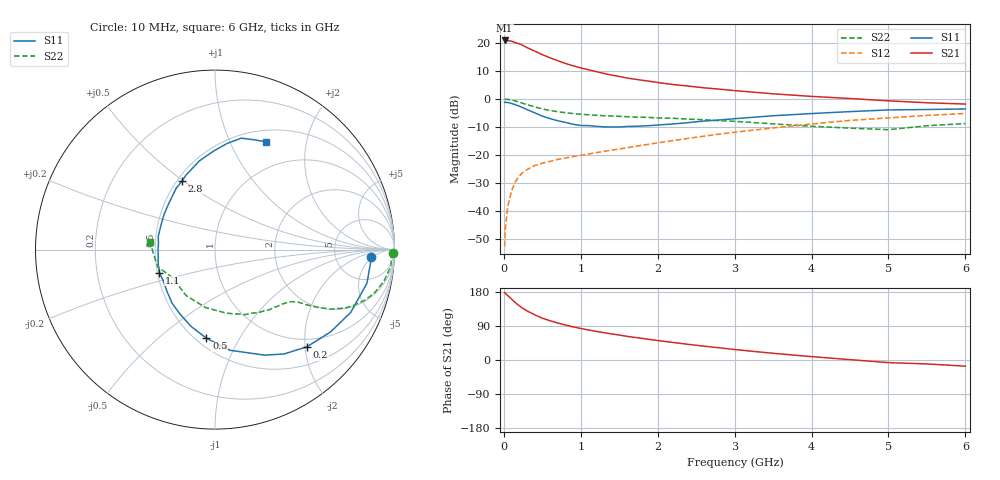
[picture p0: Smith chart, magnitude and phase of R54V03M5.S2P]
! SIEMENS Small Signal Semiconductors
! BFR183
! Si NPN RF Bipolar Junction Transistor in SOT23
! VCE = 4 V  IC = 3.5 mA
! Common Emitter S-Parameters:  May  1996
# GHz  S  MA  R  50
!  f  S11  S21  S12  S22
! GHz  MAG  ANG  MAG  ANG  MAG  ANG  MAG  ANG
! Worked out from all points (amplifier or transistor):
!   36 points, 10 MHz to 6 GHz, reference 50 ohm
!   highest |S21| = 20.8 dB at 10 MHz (marker M1)
!   |S21| within 3 dB of that: start of sweep to 337.5 MHz
!   unconditionally stable (mu >= 1): 1.211 GHz to 2.683 GHz
!   at 250 MHz: K = 0.33, MSG = 22.6 dB, |S12| = -26.1 dB
!   at 1.4 GHz: K = 1.05, MAG = 12.0 dB, |S12| = -18.2 dB
!   at 6 GHz: K = 0.88, MSG = 1.7 dB, |S12| = -5.2 dB
!   S11 on the Smith chart (normalised r, x): 10 MHz: 13, -4; 200 MHz: 0.84, -2.04; 500 MHz: 0.56, -0.74; 1.1 GHz: 0.51, -0.15; 2.8 GHz: 0.53, +0.49; 6 GHz: 0.64, +1.38
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0.01  0.8713 -2.6  11 178.2  0.0024 87.6  0.9932 -1.1
0.02  0.8698 -4.9  10.8 175.9  0.005 87.3  0.9833 -2.1
0.05  0.867 -12.5  10.9 170.2  0.0118 82.9  0.9842 -5.4
0.1  0.8333 -24.8  10.69 160.8  0.0233 77.3  0.9582 -10.5
0.15  0.7905 -35.5  10.04 151.3  0.0336 71.2  0.9224 -15.0
0.2  0.7453 -46.6  9.587 143.3  0.0422 66.9  0.8824 -18.6
0.25  0.6974 -56.5  8.943 135.9  0.0495 62.1  0.8341 -21.8
0.3  0.6494 -64.9  8.214 129.7  0.0553 59.7  0.7947 -24.2
0.4  0.5668 -81.6  7.125 119.5  0.0652 55.2  0.725 -27.2
0.5  0.4961 -95.5  6.15 110.4  0.072 52.4  0.6656 -29.1
0.6  0.4479 -107.4  5.405 103.6  0.0778 51.5  0.6227 -30.3
0.7  0.41 -118.1  4.802 97.6  0.0837 51.1  0.5944 -31.1
0.8  0.3826 -128.6  4.287 92.2  0.0889 50.7  0.5693 -31.7
0.9  0.3553 -138.7  3.898 87.4  0.0945 51.2  0.5505 -32.2
1.1  0.3355 -157.5  3.31 79.3  0.1047 52.7  0.5227 -33.8
1.6  0.3243 167.1  2.363 62.5  0.1355 55.1  0.4836 -38.7
2.2  0.3591 137.2  1.806 46.3  0.1814 56.1  0.4532 -47.5
2.8  0.4225 115.9  1.496 32.2  0.2369 53.5  0.4105 -59.5
3.5  0.503 99.8  1.236 17.7  0.3049 47.4  0.3602 -79.7
4.5  0.5957 83.4  1.019 1.0  0.4154 35.7  0.3026 -122.1
5.5  0.6497 70.3  0.856 -10.4  0.5094 22.7  0.3339 -163.5
6  0.6646 64.7  0.812 -16.3  0.5522 14.2  0.3651 173.4
